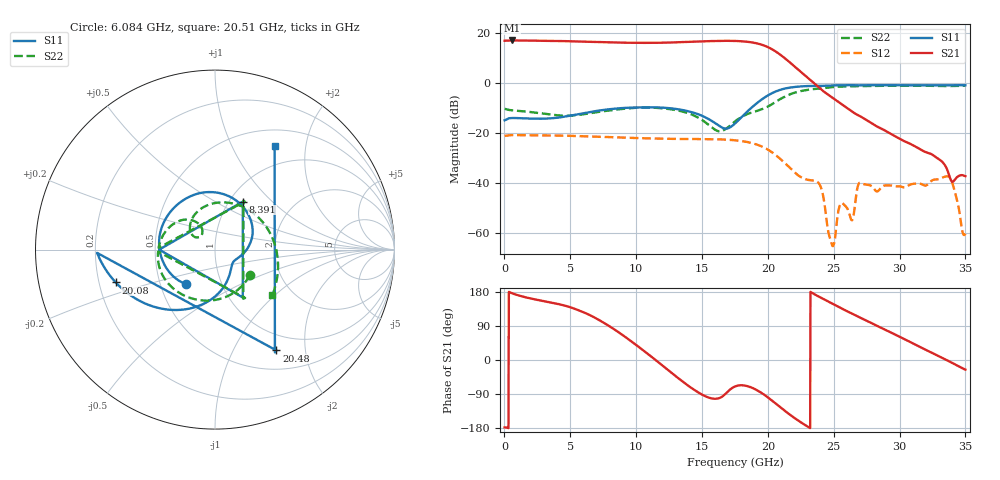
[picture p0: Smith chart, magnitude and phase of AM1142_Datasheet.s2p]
!Keysight Technologies,N5245B,MY58422270,A.16.20.02
!Date: Friday, June 9, 2023 09:41:41
!Correction: S11(C  2-Port  )
!S12(C  2-Port  )
!S21(C  2-Port  )
!S22(C  2-Port  )
!S2P File: Measurements: S11, S21, S12, S22:
# Hz S  dB  R 50
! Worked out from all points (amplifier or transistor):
!   6401 points, 10 MHz to 35 GHz, reference 50 ohm
!   highest |S21| = 17.0 dB at 556.7 MHz (marker M1)
!   |S21| within 3 dB of that: start of sweep to 20.14 GHz
!   unconditionally stable (mu >= 1): 327.7 MHz to 6.838 GHz; 10.76 GHz to 11.84 GHz; 11.92 GHz to end of sweep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
!   at 5.838 GHz: K = 1.02, MAG = 17.9 dB, |S12| = -21.2 dB
!   at 17.5 GHz: K = 1.22, MAG = 17.0 dB, |S12| = -22.8 dB
!   at 35 GHz: K = 1470.62, MAG = -23.2 dB, |S12| = -60.1 dB
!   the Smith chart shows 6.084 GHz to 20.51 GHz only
!   S11 on the Smith chart (normalised r, x): 6.084 GHz: 0.68, -0.28; 8.391 GHz: 1.15, +0.68; 20.08 GHz: 0.27, -0.15; 20.48 GHz: 0.76, -1.50; 20.51 GHz: 0.72, +1.48
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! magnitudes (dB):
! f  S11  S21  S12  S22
! 10 MHz  -14.9  16.9  -21.1  -10.3
! 556.7 MHz  -14.0  17.0  -20.8  -10.9
! 5.843 GHz  -12.2  16.5  -21.2  -12.6
! 6.084 GHz  -12.0  16.5  -21.3  -12.4
! 8.391 GHz  -10.2  16.2  -21.6  -10.7
! 11.68 GHz  -9.7  16.1  -22.2  -9.9
! 16.26 GHz  -16.9  16.8  -22.4  -19.2
! 17.5 GHz  -16.1  16.8  -22.8  -15.3
! 20.08 GHz  -4.7  14.1  -26.8  -9.2
! 20.48 GHz  -3.6  13.0  -28.3  -7.9
! 20.51 GHz  -3.6  12.9  -28.4  -7.8
! 23.34 GHz  -1.2  0.7  -38.8  -2.5
! 24.04 GHz  -1.1  -2.5  -41.8  -2.1
! 24.63 GHz  -1.0  -4.9  -60.4  -1.7
! 24.91 GHz  -0.9  -5.9  -65.0  -1.6
! 25.5 GHz  -0.9  -8.1  -48.4  -1.4
! 26.39 GHz  -0.8  -11.4  -54.7  -1.3
! 26.97 GHz  -0.9  -13.1  -39.8  -1.3
! 29.17 GHz  -0.9  -19.8  -40.8  -1.1
! 32.6 GHz  -0.9  -29.0  -38.5  -1.1
! 33.72 GHz  -0.9  -36.0  -37.3  -1.2
! 35 GHz  -0.9  -37.2  -60.1  -1.1
